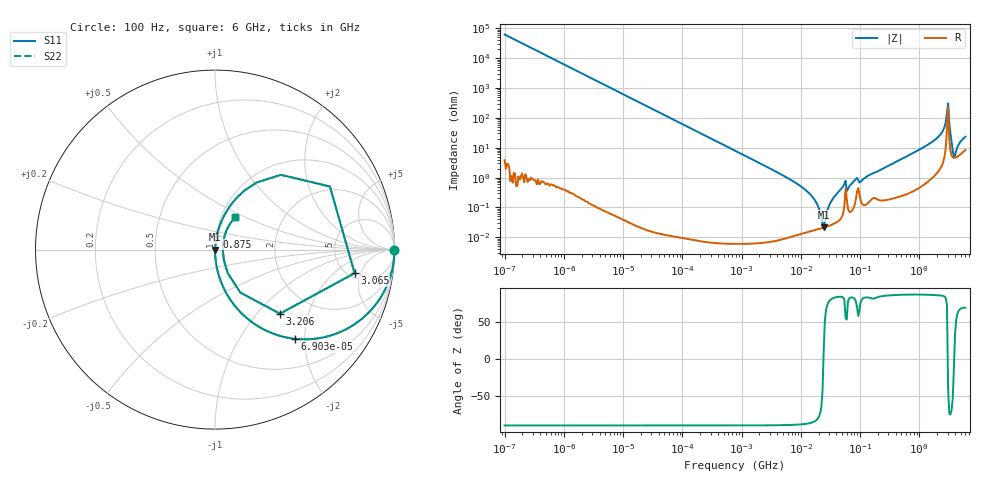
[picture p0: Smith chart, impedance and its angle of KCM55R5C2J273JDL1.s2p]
!Murata Part Number: KCM55R5C2J273JDL1
!These Parameters are Measured in Series Mode Connection
!Data Generated on Mar 13, 2026
!  o--ll--o
!Port1  Port2
!  o------o
!Operation Temp=25[degC], DC Bias Voltage=0[V]
!Freq. Start=100[Hz] Stop=6[GHz] 401[Steps]
# Hz S RI R 50
!Freq.(Hz) S11(Real) S11(Imag) S21(Real) S21(Imag) S12(Real) S12(Imag) S22(Real) S22(Imag)
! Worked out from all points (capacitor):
!   401 points, 100 Hz to 6 GHz, reference 50 ohm
!   read as one part in series: C = 25.7 nF near 109 Hz
!   lowest |Z| = 21.6 mohm at 24.34 MHz (marker M1)
!   series resonance near 24.14 MHz, so ESL is about 1.7 nH
!   S11 on the Smith chart (normalised r, x): 100 Hz: open; 69.03 kHz: 1.00, -1.80; 875 MHz: 1.01, +0.15; 3.065 GHz: 5.67, -3.94; 3.206 GHz: 1.39, -1.33; 6 GHz: 1.17, +0.44
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100  1 -0.00161  2.7e-06 0.00161  2.7e-06 0.00161  1 -0.00161
2008  0.999 -0.0323  0.00105 0.0323  0.00105 0.0323  0.999 -0.0323
14402  0.9488 -0.2203  0.0512 0.2203  0.0512 0.2203  0.9488 -0.2203
40335  0.7028 -0.457  0.2972 0.457  0.2972 0.457  0.7028 -0.457
69028  0.4467 -0.4971  0.5533 0.4971  0.5533 0.4971  0.4467 -0.4971
184852  0.1013 -0.3015  0.8987 0.3015  0.8987 0.3015  0.1013 -0.3015
774597  0.00642 -0.0795  0.9936 0.0795  0.9936 0.0795  0.00642 -0.0795
6948629  0.000171 -0.00815  0.9998 0.00815  0.9998 0.00815  0.000171 -0.00815
1.555665e7  0.000171 -0.00231  0.9998 0.00231  0.9998 0.00231  0.000171 -0.00231
2.434276e7  0.000211 4.28e-05  0.9998 -4.28e-05  0.9998 -4.28e-05  0.000211 4.28e-05
3.184506e7  0.000257 0.00145  0.9997 -0.00145  0.9997 -0.00145  0.000257 0.00145
5.211241e7  0.000688 0.00518  0.9993 -0.00518  0.9993 -0.00518  0.000688 0.00518
6.518806e7  0.000754 0.00487  0.9992 -0.00487  0.9992 -0.00487  0.000754 0.00487
3.124326e8  0.00253 0.0258  0.9975 -0.0258  0.9975 -0.0258  0.00253 0.0258
8.749838e8  0.00934 0.0736  0.9907 -0.0736  0.9907 -0.0736  0.00934 0.0736
2.142435e9  0.0694 0.2212  0.9306 -0.2212  0.9306 -0.2212  0.0694 0.2212
2.679998e9  0.2322 0.3739  0.7678 -0.3739  0.7678 -0.3739  0.2322 0.3739
3.065283e9  0.7778 -0.1314  0.2222 0.1314  0.2222 0.1314  0.7778 -0.1314
3.205649e9  0.3617 -0.357  0.6383 0.357  0.6383 0.357  0.3617 -0.357
3.666503e9  0.0496 -0.06  0.9504 0.06  0.9504 0.06  0.0496 -0.06
4.009986e9  0.0449 0.0276  0.9551 -0.0276  0.9551 -0.0276  0.0449 0.0276
6e9  0.1134 0.1794  0.8866 -0.1794  0.8866 -0.1794  0.1134 0.1794
